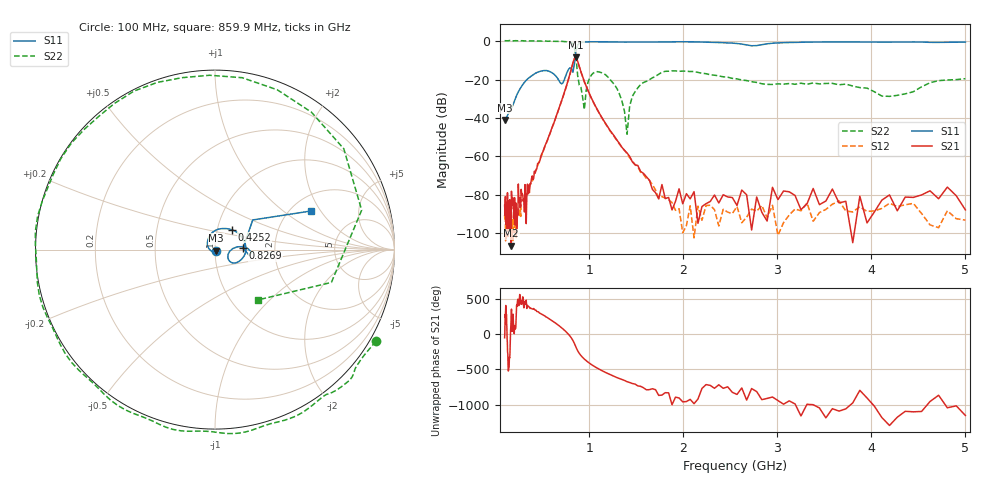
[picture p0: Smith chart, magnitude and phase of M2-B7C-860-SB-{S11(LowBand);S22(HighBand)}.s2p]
!Agilent Technologies,N5230A,MY45001737,A.07.50.48
!Agilent N5230A: A.07.50.48
!Date: Saturday, August 12, 2023 10:13:54
!Correction: S11(Full 2 Port(1,4))
!S41(Full 2 Port(1,4))
!S14(Full 2 Port(1,4))
!S44(Full 2 Port(1,4))
!S2P File: Measurements: S11, S41, S14, S44:Log Frequency Sweep
# Hz S  MA  R 50
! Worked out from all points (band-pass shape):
!   201 points, 100 MHz to 5 GHz, reference 50 ohm
!   highest |S21| = -8.48 dB at 859.9 MHz (marker M1); lowest = -106.4 dB at 169.6 MHz (marker M2)
!   |S21| within 3 dB of the highest: 825.5 MHz to 883.6 MHz (58.09 MHz wide, 6.8 % of centre)
!   lowest |S11| = -41.0 dB at 100 MHz (marker M3), VSWR 1.02, Z = 50.7 - j0.528 ohm
!   |S11| at or under -10 dB: start of sweep to 846.8 MHz
!   |S22| runs from -48.4 to 0.4 dB; largest |S21 - S12| = 0.012
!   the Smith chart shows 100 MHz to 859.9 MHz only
!   S11 on the Smith chart (normalised r, x): 100 MHz: 1.01, -0.01; 425.2 MHz: 1.17, +0.27; 826.9 MHz: 1.37, +0.02; 859.9 MHz: 2.55, +1.64
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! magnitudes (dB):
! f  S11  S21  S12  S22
! 100 MHz  -41.0  -85.5  -90.5  0.3
! 169.6 MHz  -35.2  -106.4  -86.6  0.2
! 245.9 MHz  -26.4  -74.3  -87.5  0.2
! 250.8 MHz  -25.9  -82.2  -89.0  0.2
! 349.7 MHz  -19.4  -79.5  -77.0  0.2
! 425.2 MHz  -16.8  -68.7  -68.1  0.1
! 707.1 MHz  -22.2  -30.9  -31.0  -0.1
! 826.9 MHz  -16.1  -11.2  -11.5  -1.4
! 859.9 MHz  -4.8  -8.5  -8.8  -8.6
! 929.9 MHz  -0.6  -18.5  -18.8  -29.3
! 948.2 MHz  -0.5  -21.0  -21.3  -35.6
! 986 MHz  -0.3  -25.6  -25.7  -21.4
! 1.046 GHz  -0.3  -31.9  -32.1  -16.5
! 1.176 GHz  -0.3  -43.0  -43.2  -17.6
! 1.322 GHz  -0.4  -53.3  -53.7  -27.7
! 1.402 GHz  -0.5  -58.2  -58.6  -48.4
! 1.458 GHz  -0.5  -62.8  -62.4  -28.7
! 1.739 GHz  -0.4  -82.1  -81.7  -17.2
! 2.571 GHz  -1.2  -85.5  -86.0  -19.6
! 3.381 GHz  -0.5  -76.7  -93.7  -21.7
! 4.193 GHz  -0.5  -80.0  -84.4  -28.7
! 5 GHz  -0.5  -87.8  -93.1  -19.5
